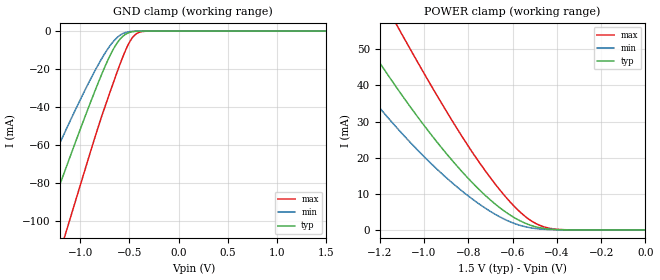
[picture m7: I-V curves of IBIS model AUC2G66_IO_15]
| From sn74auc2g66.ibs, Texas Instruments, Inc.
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[Model]   AUC2G66_IO_15
Model_type  Terminator
| variable   typ   min   max
C_comp   3.67pF   3.26pF   3.81pF
| C_tri-state   3.67pF   3.26pF   3.81pF
[Temperature Range]   40   100   -40
| Ambient temperature   25   85   -40
[Voltage range]   1.5   1.4   1.6
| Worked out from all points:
|   GND clamp passes 1 mA (typ) near -0.51 V on its own axis
|   POWER clamp passes 1 mA (typ) near -0.50 V on its own axis
[GND Clamp]
| AUC2G66_IO_15
|   Voltage   I(typ)   I(min)   I(max)
-2.7V     -295.9mA   -240.2mA   -365.2mA
-1.6V     -137.3mA   -105.1mA   -182.9mA
-1.39V    -107.1mA   -80.18mA   -147.6mA
-1.35V    -101.3mA   -75.5mA    -140.8mA
-1.145V   -72.11mA   -52.07mA   -106mA
-915mV    -40.21mA   -27.38mA   -66.86mA
-750mV    -18.95mA   -11.84mA   -40.11mA
-650mV    -8.356mA   -4.727mA   -25.29mA
-565mV    -2.697mA   -1.274mA   -13.39mA
-465mV    -326.8uA   -131.1uA   -3.206mA
-360mV    -17.59uA   -8.514uA   -188.7uA
1.5V      417.2pA    9.152nA    305.4pA
[POWER Clamp]
| AUC2G66_IO_15
|   Voltage   I(typ)   I(min)   I(max)
-2.7V     212.8mA    183.5mA    242.9mA
-1.475V   73.08mA    55.64mA    96.87mA
-1.305V   56.19mA    41.71mA    77.24mA
-1.28V    53.79mA    39.77mA    74.39mA
-1.12V    39.12mA    28.13mA    56.42mA
-1.1V     37.37mA    26.77mA    54.22mA
-935mV    23.87mA    16.48mA    36.58mA
-780mV    12.99mA    8.49mA     21.35mA
-645mV    5.579mA    3.233mA    10.17mA
-540mV    1.802mA    857.8uA    3.612mA
-400mV    105.1uA    48.24uA    194.6uA
-35.59fV  417.2pA    755.8pA    349.3pA
